TYPE SimuParameter :
STRUCT
	cClampAtWork				: LREAL	:= 3.0;				// 正位气缸目标位置的坐标
	cClampAtBase				: LREAL	:= 0.0;				// 正位气缸基始位置的坐标
	cBarrierAtWork				: LREAL	:= 63.0;			// 栏杆气缸目标位置的坐标
	cBarrierAtBase				: LREAL	:= 0.0;				// 栏杆气缸基始位置的坐标
	cMetalAtWorkMin				: LREAL	:= -72.9;			// 金属分拣气缸在工作位置的上限坐标
	cMetalAtWorkMax				: LREAL	:= -73.1;			// 金属分拣气缸在工作位置的下限坐标
	cMetalAtBase				: LREAL	:= 0.0;				// 金属分拣气缸在基始位置的坐标
	cPlasticAtWorkMin			: LREAL	:= -72.9;			// 塑料分拣气缸在工作位置的上限坐标
	cPlasticAtWorkMax			: LREAL	:= -73.1;			// 塑料分拣气缸在工作位置的下限坐标
	cPlasticAtBase				: LREAL	:= 0.0;				// 塑料分拣气缸在基始位置的坐标
	

	cSensorsBoxesY				: LREAL	:= -5.0;			// 正常运输时的纵坐标
	cBarrierSensorBox1Xmin		: LREAL	:= -1.0;			// 栏杆前传感器检测到物料1的下限坐标
	cBarrierSensorBox1Xmax		: LREAL	:= 60.0;			// 栏杆前传感器检测到物料1的上限坐标
	cBarrierSensorBox2Xmin		: LREAL	:= 59.0;			// 栏杆前传感器检测到物料2的下限坐标
	cBarrierSensorBox2Xmax		: LREAL	:= 120.0;			// 栏杆前传感器检测到物料2的上限坐标
	cBarrierSensorBox3Xmin		: LREAL := 119.0;			// 栏杆前传感器检测到物料3的下限坐标
	cBarrierSensorBox3Xmax		: LREAL := 180.0;			// 栏杆前传感器检测到物料3的下限坐标
	cBarrierSensorBox4Xmin		: LREAL := 179.0;			// 栏杆前传感器检测到物料4的上限坐标
	cBarrierSensorBox4Xmax		: LREAL := 240.0;			// 栏杆前传感器检测到物料5的下限坐标
	
	cMetalSensorBox1Xmin		: LREAL := 134.0;			// 金属物料传感器检测到物料1的下限坐标
	cMetalSensorBox1Xmax		: LREAL := 197.0;			// 金属物料传感器检测到物料1的上限坐标
	cMetalSensorBox2Xmin		: LREAL := 194.0;			// 金属物料传感器检测到物料2的下限坐标
	cMetalSensorBox2Xmax		: LREAL := 257.0;			// 金属物料传感器检测到物料2的上限坐标
	cMetalSensorBox3Xmin		: LREAL := 254.0;			// 金属物料传感器检测到物料3的下限坐标	
	cMetalSensorBox3Xmax		: LREAL := 317.0;			// 金属物料传感器检测到物料3的上限坐标
	cMetalSensorBox4Xmin		: LREAL := 314.0;			// 金属物料传感器检测到物料4的下限坐标
	cMetalSensorBox4Xmax		: LREAL := 377.0;			// 金属物料传感器检测到物料4的上限坐标
	
	cPlasticSensorBox1Xmin		: LREAL := 384.0;			// 塑料物料传感器检测到物料1的下限坐标
	cPlasticSensorBox1Xmax		: LREAL := 447.0;			// 塑料物料传感器检测到物料1的上限坐标
	cPlasticSensorBox2Xmin		: LREAL := 444.0;			// 塑料物料传感器检测到物料2的下限坐标
	cPlasticSensorBox2Xmax		: LREAL := 507.0;			// 塑料物料传感器检测到物料2的上限坐标
	cPlasticSensorBox3Xmin		: LREAL := 504.0;			// 塑料物料传感器检测到物料3的下限坐标
	cPlasticSensorBox3Xmax		: LREAL := 567.0;			// 塑料物料传感器检测到物料3的上限坐标
	cPlasticSensorBox4Xmin		: LREAL := 564.0;			// 塑料物料传感器检测到物料4的下限坐标
	cPlasticSensorBox4Xmax		: LREAL := 627.0;			// 塑料物料传感器检测到物料4的上限坐标
	
	cClampTempMax				: LREAL := 60.5;			// 正位气缸最大设定温度
	cClampTempMin				: LREAL := 9.4;				// 正位气缸最小设定温度
	cClampTempCurrent			: LREAL := 10.7;			// 正位气缸当前温度
	
	cBarrierTempMax				: LREAL := 55.0;			// 栏杆气缸最大设定温度
	cBarrierTempMin				: LREAL := 10.0;			// 栏杆气缸最小设定温度
	cBarrierTempChange			: LREAL := 1.2;				// 栏杆气缸的温度变化值
	

END_STRUCT
END_TYPE
